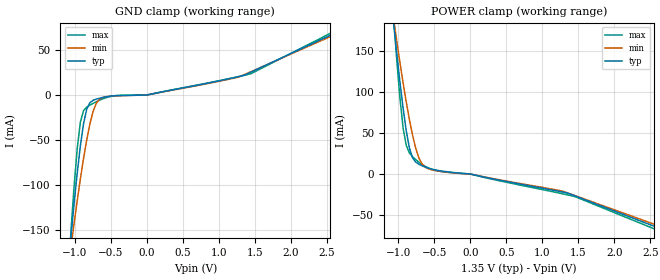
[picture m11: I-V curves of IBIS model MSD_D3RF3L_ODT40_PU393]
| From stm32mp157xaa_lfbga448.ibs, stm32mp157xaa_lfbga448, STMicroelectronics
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[Model] MSD_D3RF3L_ODT40_PU393
Model_type   Input
C_comp 2.304pF   2.264pF   2.357pF
Vinh = 810.000mV
Vinl = 540.000mV
[Temperature Range]   25.000   125.000   -40.000
[Voltage Range]   1.350V   1.283V   1.450V
[GND Clamp Reference]   0.00V   0.00V   0.00V
[POWER Clamp Reference]   1.350V   1.283V   1.450V
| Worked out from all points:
|   GND clamp passes 1 mA (typ) near -0.47 V on its own axis
|   POWER clamp passes 1 mA (typ) near -0.14 V on its own axis
[GND Clamp]
-1.318V   -415.1mA   -341mA     -533mA
-1.055V   -159mA     -170.3mA   -153mA
-1.011V   -121.4mA   -143.5mA   -102.4mA
-966.7mV  -86.93mA   -117.8mA   -59.6mA
-922.7mV  -56.51mA   -93.28mA   -29.99mA
-878.8mV  -31.9mA    -70.58mA   -17.36mA
-834.9mV  -15.78mA   -49.99mA   -13.42mA
-747mV    -5.886mA   -18.44mA   -9.318mA
-615.1mV  -2.752mA   -2.762mA   -4.406mA
200nV     3.399nA    3.255nA    3.442nA
1.45V     25.61mA    26.04mA    23.83mA
2.68V     71.42mA    69.67mA    74.01mA
[Power Clamp]
-1.33V    440.8mA    363.4mA    565.6mA
-1.067V   184.9mA    190.1mA    192.2mA
-1.023V   147.6mA    162.9mA    140mA
-978.8mV  112.8mA    136.6mA    93.19mA
-934.9mV  80.71mA    111.6mA    56.41mA
-890.9mV  52.84mA    88.24mA    35.02mA
-847mV    31.71mA    66.75mA    25.73mA
-759.1mV  14.59mA    31.52mA    17.6mA
-671.2mV  10.08mA    12.18mA    11.76mA
-583.3mV  7.175mA    6.393mA    7.323mA
1.438V    -26.33mA   -25.92mA   -27.29mA
2.668V    -67.83mA   -65.18mA   -71.22mA
